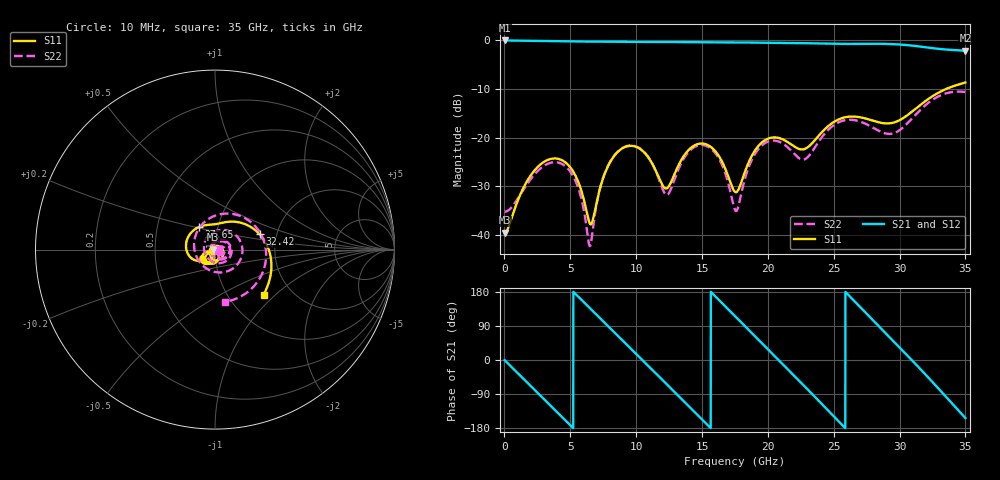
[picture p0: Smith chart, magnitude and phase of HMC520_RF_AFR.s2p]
! Analog Devices, Inc.
! 1 Analog Way
! Wilmington, MA 01887
! http://www.analog.com
! Date:  2021-09-07 NN
! Board Name:  EV1HMC520ALC4 Revision A with HMC520ALC4 installed
! File Description:  Automatic Fixture Removal S-Parameters for RF Port connector and board loss de-embedding
! File Generation:  Calibrated Network Analyzer
! Chip Part Number:  HMC520A
! Chip Description:  GaAs, MMIC, IQ Mixer
! Chip Frequency:  6 to 10 GHz
! Chip Package:  LCC, 3.9 x 3.9 x 0.9 mm
! RF Port:  HMC520ALC4 removed and end of trace left open
!Note:
!  Analog Devices supplies this data as a sample of measured data at the evaluation board
!  ports for this product.  Your particular data for this product may vary.
!  Analog Devices reserves the right to change this data at anytime.
!  All lines below in this file are as is from the Network Analyzer.
!Agilent Technologies,N5245A,MY52451809,A.10.47.06
!Automatic Fixture Removal (AFR)
!Date: Friday, August 27, 2021 5:01:42 AM
!S2P File: Measurements: S11,S21,S12,S22:
# MHz S  RI  R 50
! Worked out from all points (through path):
!   3500 points, 10 MHz to 35 GHz, reference 50 ohm
!   highest |S21| = 0.00 dB at 10 MHz (marker M1); lowest = -2.1 dB at 35 GHz (marker M2)
!   group delay of S21, straight-line fit = 97.3 ps
!   lowest |S11| = -39.5 dB at 10 MHz (marker M3), VSWR 1.02, Z = 49 + j0.0287 ohm
!   |S11| at or under -10 dB: start of sweep to 33.51 GHz
!   |S22| runs from -42.3 to -10.5 dB; largest |S21 - S12| = 1.4e-15
!   S11 on the Smith chart (normalised r, x): 10 MHz: 0.98, +0.00; 27.65 GHz: 0.81, +0.21; 32.42 GHz: 1.63, +0.30; 35 GHz: 1.45, -0.85
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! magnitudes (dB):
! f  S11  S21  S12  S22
! 10 MHz  -39.5  0.0  0.0  -35.2
! 1.68 GHz  -29.1  -0.1  -0.1  -29.7
! 3.13 GHz  -24.7  -0.1  -0.1  -25.5
! 4.73 GHz  -25.3  -0.2  -0.2  -26.1
! 5.85 GHz  -31.0  -0.2  -0.2  -32.6
! 6.49 GHz  -37.7  -0.2  -0.2  -42.3
! 7.42 GHz  -28.9  -0.3  -0.3  -28.8
! 8.62 GHz  -22.9  -0.3  -0.3  -22.8
! 10.27 GHz  -22.2  -0.3  -0.3  -22.1
! 11.68 GHz  -27.9  -0.3  -0.3  -28.2
! 12.39 GHz  -30.3  -0.3  -0.3  -31.7
! 13.89 GHz  -22.8  -0.4  -0.4  -23.2
! 15.34 GHz  -21.4  -0.4  -0.4  -21.7
! 16.48 GHz  -24.7  -0.4  -0.4  -25.3
! 17.51 GHz  -31.1  -0.4  -0.4  -34.8
! 19.67 GHz  -20.7  -0.5  -0.5  -21.3
! 23.34 GHz  -21.2  -0.6  -0.6  -22.9
! 25.38 GHz  -16.2  -0.7  -0.7  -16.8
! 27.65 GHz  -16.2  -0.7  -0.7  -17.4
! 29.17 GHz  -17.0  -0.7  -0.7  -19.2
! 32.42 GHz  -11.6  -1.6  -1.6  -12.3
! 35 GHz  -8.6  -2.1  -2.1  -10.6
